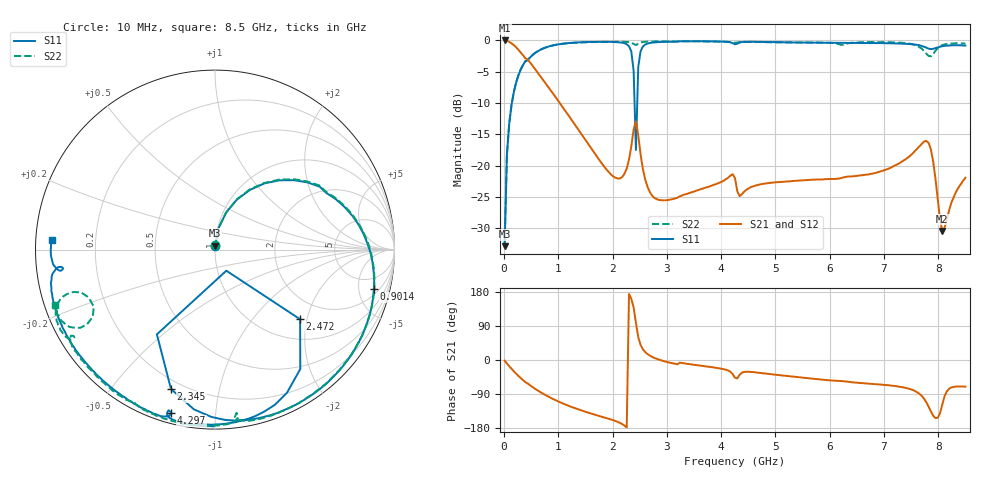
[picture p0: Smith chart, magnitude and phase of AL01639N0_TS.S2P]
!AVX CORPORATION
!PART NUMBER AL01639N0_TS
!DESCRIPTION: AIR CORE INDUCTOR, 39nH, 6 TURNS
!Agilent Technologies,E5071C,MY46102230,A.09.54
!Date: Mon Sep 03 16:33:06 2012
!Data & Calibration Information:
!Freq	S11:SOLT2(ON)	S21:SOLT2(ON)	S12:SOLT2(ON)	S22:SOLT2(ON)
# Hz S dB R 50
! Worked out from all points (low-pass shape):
!   201 points, 10 MHz to 8.5 GHz, reference 50 ohm
!   highest |S21| = -0.01 dB at 10 MHz (marker M1); lowest = -30.4 dB at 8.075 GHz (marker M2)
!   |S21| within 3 dB of the highest: start of sweep to 429.2 MHz
!   lowest |S11| = -32.9 dB at 10 MHz (marker M3), VSWR 1.05, Z = 50 + j2.28 ohm
!   |S11| at or under -10 dB: start of sweep to 143.8 MHz; 2.405 GHz to 2.454 GHz (49.16 MHz wide, 2.02 % of centre)
!   |S22| runs from -32.7 to -0.1 dB; largest |S21 - S12| = 0.011
!   S11 on the Smith chart (normalised r, x): 10 MHz: 1.00, +0.05; 901.5 MHz: 2.71, -7.14; 2.345 GHz: 0.16, -0.72; 2.472 GHz: 1.46, -1.82; 4.297 GHz: 0.05, -0.77; 8.5 GHz: 0.05, +0.03
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1e7  -32.85 88.4  -0.01 -1.7  0.07 -1.3  -32.73 89.9
5.245e7  -18.27 80.5  -0.08 -9.1  -0.05 -9.1  -18.22 80.5
1.798e8  -8.25 59.5  -0.75 -29.8  -0.74 -29.8  -8.22 59.9
5.6185e8  -2.07 13.9  -4.46 -75.1  -4.45 -75.2  -2.05 14.4
9.0145e8  -0.80 -14.0  -8.48 -102.8  -8.47 -102.9  -0.79 -13.5
1.4533e9  -0.29 -46.5  -15.31 -134.5  -15.30 -134.6  -0.31 -46.1
2.09005e9  -0.28 -77.6  -22.04 -163.1  -22.02 -163.1  -0.22 -72.6
2.34475e9  -1.78 -107.5  -16.91 161.6  -16.89 161.5  -0.35 -81.9
2.3872e9  -4.84 -124.4  -14.22 138.6  -14.21 138.5  -0.55 -83.2
2.42965e9  -17.49 -61.7  -12.88 98.2  -12.87 98.1  -0.75 -82.5
2.4721e9  -4.26 -39.3  -15.13 60.6  -15.13 60.6  -0.51 -82.0
2.51455e9  -1.75 -54.5  -18.15 40.1  -18.15 40.0  -0.35 -83.3
2.59945e9  -0.66 -68.9  -22.17 21.1  -22.17 21.1  -0.22 -86.1
2.85415e9  -0.27 -84.9  -25.48 1.0  -25.50 1.1  -0.16 -93.0
3.19375e9  -0.21 -96.2  -25.13 -11.3  -25.11 -11.2  -0.14 -100.6
4.255e9  -0.62 -106.1  -21.99 -46.8  -21.98 -46.8  -0.38 -118.0
4.29745e9  -0.53 -105.0  -24.09 -48.4  -24.10 -48.3  -0.33 -118.3
5.6983e9  -0.36 -131.6  -22.23 -49.5  -22.26 -49.6  -0.35 -143.1
7.09915e9  -0.45 -159.7  -20.43 -66.9  -20.42 -67.0  -0.29 -155.8
7.8208e9  -1.32 -173.5  -16.34 -122.6  -16.33 -122.7  -2.47 -159.3
8.0755e9  -0.93 -174.1  -30.44 -116.9  -30.51 -116.7  -0.74 -152.1
8.5e9  -0.82 176.5  -21.93 -70.3  -21.91 -70.3  -0.52 -160.9
